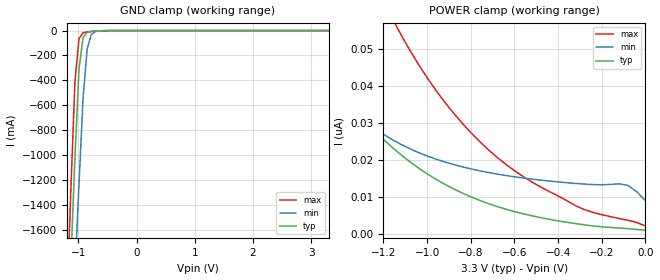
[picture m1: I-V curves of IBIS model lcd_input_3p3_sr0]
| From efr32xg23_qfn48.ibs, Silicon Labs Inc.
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|   Model lcd_input_3p3_sr0
[Model]  lcd_input_3p3_sr0
Model_type Input
C_comp   1.6300pF   1.4000pF   2.7000pF
[Temperature Range]   25.0000   0.1250k   -40.0000
[Pullup Reference]   3.3000V   3.0000V   3.6000V
[Pulldown Reference]   0.0V   0.0V   0.0V
[POWER Clamp Reference]   3.3000V   3.0000V   3.6000V
[GND Clamp Reference]   0.0V   0.0V   0.0V
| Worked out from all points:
|   GND clamp passes 1 mA (typ) near -0.56 V on its own axis
[GND_clamp]
|Voltage   I(typ)   I(min)   I(max)
-3.3V     -27.87A    -25.05A    -30.64A
-1.2V     -2.686A    -3.389A    -2.22A
-1.13V    -1.852A    -2.669A    -1.282A
-1.06V    -1.021A    -1.951A    -413.8mA
-990mV    -311.8mA   -1.235A    -64.72mA
-920mV    -56.25mA   -542.5mA   -17.8mA
-850mV    -13.45mA   -148.5mA   -11.08mA
-780mV    -6.591mA   -32.68mA   -7.457mA
-710mV    -4.029mA   -8.323mA   -4.574mA
-360mV    -18.91uA   -70.05uA   -6.844uA
3.3V      1.07nA     13.64nA    781.9pA
[POWER_clamp]
|Voltage   I(typ)   I(min)   I(max)
-3.28V    727.8nA    32.99uA    1.086uA
-1.6V     57.64nA    55.6nA     128.6nA
-1.56V    53.42nA    50.92nA    120.3nA
-1.4V     38.98nA    37.13nA    91.2nA
-1.16V    23.46nA    25.56nA    58.31nA
-1.12V    21.47nA    24.28nA    53.91nA
-880mV    12.29nA    18.85nA    32.79nA
-640mV    6.783nA    15.87nA    18.92nA
-320mV    2.894nA    13.73nA    7.713nA
-120mV    1.684nA    13.64nA    4.257nA
-80mV     1.52nA     13.19nA    3.779nA
0V        1.07nA     9.091nA    2.25nA
